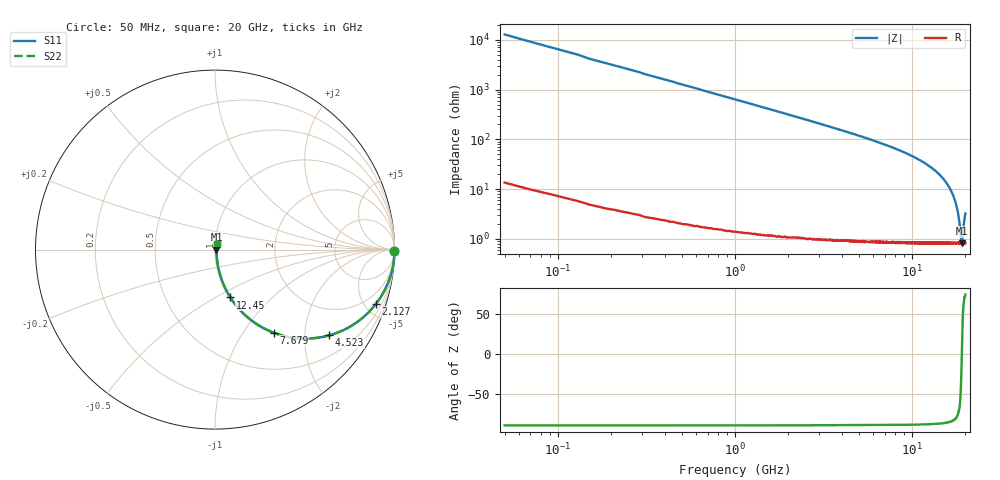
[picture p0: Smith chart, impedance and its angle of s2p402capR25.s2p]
! AVX Thin Film Operation		Date: September 2011
! Description: Accu-P® Series, Thin Film, SMD, RF Capacitor
! Part Number: 04021JR25ZBW/STR
! 50 MHz  -  20 GHz
! Serial Measurements
# MHZ S MA R 50
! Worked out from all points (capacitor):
!   1000 points, 50 MHz to 20 GHz, reference 50 ohm
!   read as one part in series: C = 251 fF near 149.8 MHz
!   lowest |Z| = 816 mohm at 19.08 GHz (marker M1)
!   series resonance near 19.07 GHz, so ESL is about 280 pH
!   S11 on the Smith chart (normalised r, x): 50 MHz: open; 2.127 GHz: 1.03, -5.91; 4.523 GHz: 1.02, -2.66; 7.679 GHz: 1.02, -1.39; 12.45 GHz: 1.02, -0.59; 20 GHz: 1.02, +0.06
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50  1 -0.5  0.007854 89.5  0.007854 89.5  1 -0.5
189.79  1 -1.7  0.03 88.2  0.03 88.2  1 -1.7
269.67  0.999 -2.4  0.042 87.5  0.042 87.5  0.999 -2.4
609.159  0.995 -5.5  0.095 84.4  0.095 84.4  0.995 -5.5
1208.258  0.982 -10.8  0.187 79.1  0.187 79.1  0.982 -10.8
2126.877  0.946 -18.7  0.32 71.1  0.32 71.1  0.946 -18.7
3384.985  0.875 -28.7  0.48 61.0  0.48 61.0  0.875 -28.7
4523.273  0.796 -36.8  0.599 52.8  0.599 52.8  0.796 -36.8
6700  0.637 -49.9  0.764 39.5  0.764 39.5  0.637 -49.9
7678.529  0.567 -54.7  0.817 34.6  0.817 34.6  0.567 -54.7
10034.99  0.414 -64.5  0.903 24.5  0.903 24.5  0.414 -64.5
12451.35  0.28 -72.2  0.952 16.2  0.952 16.2  0.28 -72.2
13350  0.235 -74.5  0.964 13.6  0.964 13.6  0.235 -74.5
15267.12  0.147 -78.4  0.981 8.5  0.981 8.5  0.147 -78.4
16684.99  0.089 -79.7  0.988 5.1  0.988 5.1  0.089 -79.7
18042.94  0.038 -75.4  0.991 2.1  0.991 2.1  0.038 -75.4
18402.4  0.025 -69.6  0.992 1.4  0.992 1.4  0.025 -69.6
18961.56  0.009088 -25.5  0.992 0.2  0.992 0.2  0.009088 -25.5
19081.38  0.008191 1.6  0.992 -0.0  0.992 -0.0  0.008191 1.6
19201.2  0.009282 27.9  0.992 -0.3  0.992 -0.3  0.009282 27.9
19660.51  0.022 66.6  0.992 -1.1  0.992 -1.1  0.022 66.6
20000  0.032 73.6  0.991 -1.8  0.991 -1.8  0.032 73.6
